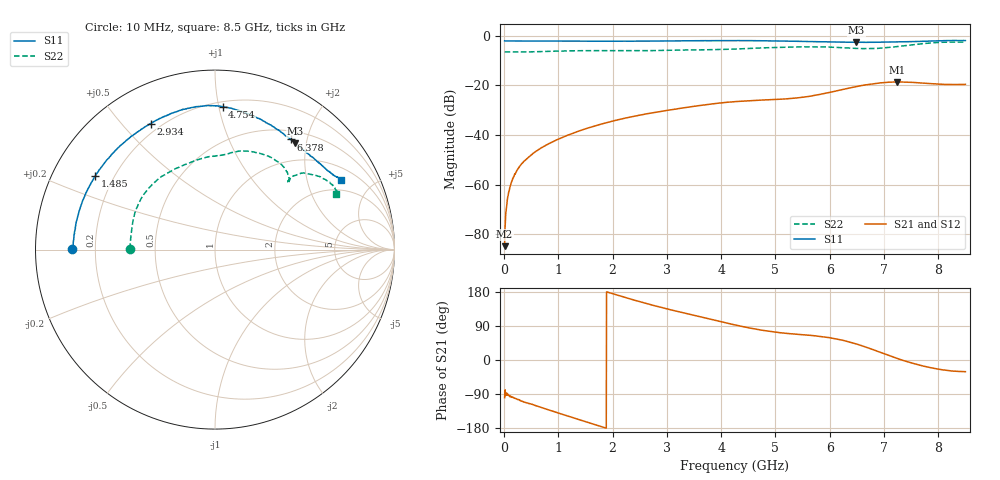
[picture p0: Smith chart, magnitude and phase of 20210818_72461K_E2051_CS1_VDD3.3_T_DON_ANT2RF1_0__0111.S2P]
!Agilent Technologies,E5071C,MY46417908,A.11.23
!Date: Wed Aug 18 14:24:44 2021
!Data & Calibration Information:
!Freq	S11:SOLT2(ON)	S21:SOLT2(ON)	S12:SOLT2(ON)	S22:SOLT2(ON)
!PortZ  Port1:50+j0  Port2:50+j0
!Above PortZ is port z conversion or system Z0 setting when saving the data.
!When reading, reference impedance value at option line is always used.
# Hz S dB R 50
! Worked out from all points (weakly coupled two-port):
!   1601 points, 10 MHz to 8.5 GHz, reference 50 ohm
!   highest |S21| = -18.57 dB at 7.248 GHz (marker M1); lowest = -84.9 dB at 10 MHz (marker M2)
!   lowest |S11| = -2.6 dB at 6.489 GHz (marker M3), VSWR 6.72, Z = 34.3 + j90 ohm
!   |S11| at or under -10 dB: nowhere
!   |S22| runs from -6.5 to -2.5 dB; largest |S21 - S12| = 0.00047
!   S11 on the Smith chart (normalised r, x): 10 MHz: 0.11, +0.00; 1.485 GHz: 0.13, +0.28; 2.934 GHz: 0.16, +0.60; 4.754 GHz: 0.24, +1.03; 6.378 GHz: 0.63, +1.73; 8.5 GHz: 1.48, +3.26
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1e7  -2.00 179.7  -84.87 -99.5  -80.63 -97.3  -6.46 179.6
7.3675e7  -2.04 178.4  -64.59 -92.5  -64.22 -93.4  -6.48 178.0
1.108188e8  -2.04 177.7  -60.94 -97.2  -60.82 -95.8  -6.49 177.0
1.957188e8  -2.06 175.8  -55.78 -101.3  -55.97 -101.0  -6.51 174.6
3.124562e8  -2.07 173.3  -51.91 -108.3  -51.86 -107.5  -6.48 171.7
5.247062e8  -2.07 168.9  -47.67 -117.5  -47.64 -117.6  -6.42 166.4
7.369562e8  -2.09 164.3  -44.59 -128.0  -44.56 -127.9  -6.30 160.5
1.426769e9  -2.12 149.7  -38.04 -159.4  -38.05 -159.4  -5.97 139.8
1.485138e9  -2.12 148.5  -37.63 -162.2  -37.64 -162.1  -5.97 138.0
2.127194e9  -2.13 134.3  -33.71 169.5  -33.72 169.5  -6.00 119.2
2.843538e9  -2.07 118.9  -30.66 140.8  -30.65 140.7  -5.88 102.6
2.933744e9  -2.06 117.0  -30.31 137.6  -30.32 137.6  -5.86 100.9
4.255e9  -1.91 94.1  -26.53 92.6  -26.53 92.5  -5.31 81.4
4.753788e9  -1.97 87.0  -25.89 78.7  -25.89 78.7  -4.86 73.7
5.671769e9  -2.29 70.7  -24.20 64.7  -24.22 64.8  -4.42 54.6
6.3775e9  -2.56 55.5  -20.96 47.1  -20.98 46.9  -4.92 43.1
6.488931e9  -2.61 53.0  -20.48 42.4  -20.50 42.3  -5.06 42.6
7.088538e9  -2.48 41.7  -18.70 12.2  -18.72 12.1  -4.66 43.5
7.247725e9  -2.42 39.2  -18.57 3.9  -18.59 3.9  -4.29 42.8
7.507731e9  -2.31 35.1  -18.74 -7.8  -18.75 -7.8  -3.62 40.2
8.011825e9  -1.99 30.2  -19.47 -24.5  -19.45 -24.6  -2.64 30.7
8.5e9  -1.90 28.9  -19.56 -30.8  -19.57 -31.0  -2.58 24.4
